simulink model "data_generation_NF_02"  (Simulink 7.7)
settings: Solver=VariableStepDiscrete  StartTime=0.0  StopTime=3000  RelTol=1e-3
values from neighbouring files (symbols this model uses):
  A = [0.9944 -0.1203 -0.4302    [process_model02.m]
  B = [1 0    [process_model02.m]
  C = [1 0 0    [process_model02.m]
  D = zeros(2,2)    [process_model02.m]
  q2 = (0.05)^2    (= 0.0025)    [process_model02.m]    (also in UIO_KF_designs.m)
  r2 = (0.6)^2    (= 0.36)    [process_model02.m]    (also in UIO_KF_designs.m)
  Ts = 0.1    [process_model02.m]
  x0 = [0.01 0.02 0.03]    [process_model02.m]
libraries: simulink x2

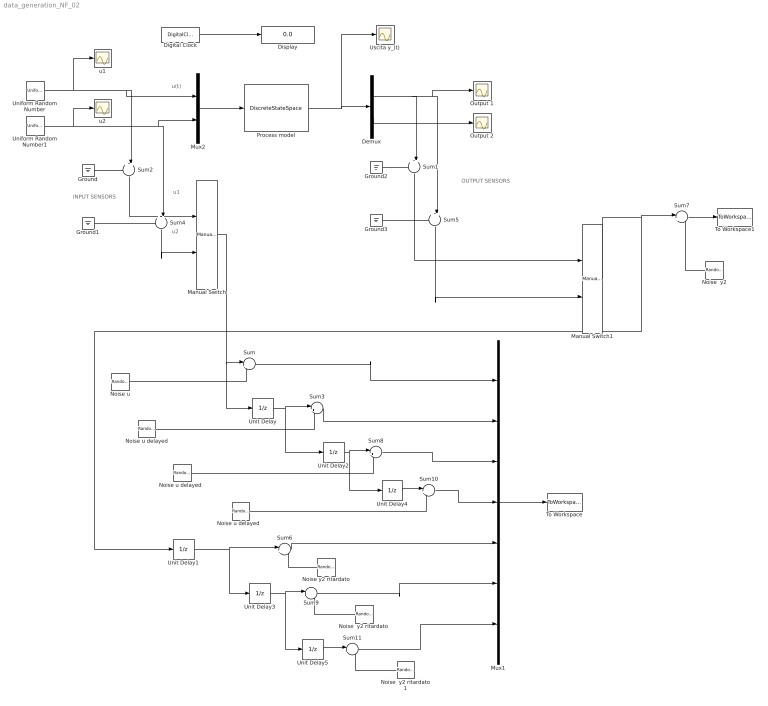
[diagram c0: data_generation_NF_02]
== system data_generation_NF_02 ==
  note: u(t)
  note: INPUT SENSORS
  note: OUTPUT SENSORS
  note: u1
  note: u2
  Demux : Demux  Outputs=2
  Digital Clock : DigitalClock  SampleTime=Ts
  Display : Display
  Ground{,1..3} (4 alike) : Ground
  Manual Switch : simulink/Signal Routing/Manual Switch  SystemSampleTime=-1  sw=1  action=0  varsize=off
  Manual Switch1 : simulink/Signal Routing/Manual Switch  SystemSampleTime=-1  sw=1  action=0  varsize=off
  Mux1 : Mux  Inputs=7
  Mux2 : Mux  Inputs=2
  Noise u : RandomNumber  Variance=q2  Seed=1  SampleTime=Ts
  Noise u delayed : RandomNumber  Variance=q2  Seed=2  SampleTime=Ts
  "Noise u delayed  " : RandomNumber  Variance=q2  Seed=17  SampleTime=Ts
  "Noise u delayed   " : RandomNumber  Variance=q2  Seed=33  SampleTime=Ts
  Noise  y2 : RandomNumber  Variance=r2  Seed=3  SampleTime=Ts
  "Noise  y2 ritardato " : RandomNumber  Variance=r2  Seed=21  SampleTime=Ts
  Noise  y2 ritardato 1 : RandomNumber  Variance=r2  Seed=44  SampleTime=Ts
  Noise y2 ritardato : RandomNumber  Variance=r2  Seed=4  SampleTime=Ts
  Output 1 : Scope
  Output 2 : Scope
  Process model : DiscreteStateSpace  A=A  B=B  C=C  D=D  X0=x0  SampleTime=Ts
  Sum{,3,6..11} (8 alike) : Sum  Inputs=|++
  Sum{1..2,4..5} (4 alike) : Sum  Inputs=++|
  To Workspace : ToWorkspace  VariableName=Psim  SampleTime=Ts  SaveFormat=Array
  To Workspace1 : ToWorkspace  VariableName=Tsim  SampleTime=Ts  SaveFormat=Array
  Uniform Random Number : UniformRandomNumber  Seed=11  SampleTime=Ts
  Uniform Random Number1 : UniformRandomNumber  Minimum=-0.5  Maximum=0.5  Seed=13  SampleTime=Ts
  Unit Delay{,1..5} (6 alike) : UnitDelay  SampleTime=Ts
  Uscita y_(t) : Scope
  u1 : Scope
  u2 : Scope
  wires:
  Digital Clock/1 -> Display/1
  Mux2/1 -> Process model/1
  Uniform Random Number/1 -> u1/1, Mux2/1, Sum2/2
  Process model/1 -> Uscita y_(t)/1, Demux/1
  Uniform Random Number1/1 -> u2/1, Mux2/2, Sum4/2
  Demux/1 -> Output 1/1, Sum5/2, Sum1/2
  Demux/2 -> Output 2/1
  Sum2/1 -> Manual Switch/1
  Sum4/1 -> Manual Switch/2
  Ground/1 -> Sum2/1
  Ground1/1 -> Sum4/1
  Manual Switch/1 -> Sum/1, Unit Delay/1
  Unit Delay/1 -> Sum3/1, Unit Delay2/1
  Noise u/1 -> Sum/2
  Noise u delayed/1 -> Sum3/2
  Sum1/1 -> Manual Switch1/1
  Sum5/1 -> Manual Switch1/2
  Unit Delay1/1 -> Sum6/1, Unit Delay3/1
  Noise y2 ritardato/1 -> Sum6/2
  Manual Switch1/1 -> Unit Delay1/1, Sum7/1
  Ground2/1 -> Sum1/1
  Ground3/1 -> Sum5/1
  Sum7/1 -> To Workspace1/1
  Noise  y2/1 -> Sum7/2
  Unit Delay2/1 -> Sum8/1, Unit Delay4/1
  "Noise u delayed  "/1 -> Sum8/2
  Mux1/1 -> To Workspace/1
  Unit Delay3/1 -> Sum9/1, Unit Delay5/1
  "Noise  y2 ritardato "/1 -> Sum9/2
  Unit Delay4/1 -> Sum10/1
  "Noise u delayed   "/1 -> Sum10/2
  Sum6/1 -> Mux1/5
  Sum10/1 -> Mux1/4
  Sum8/1 -> Mux1/3
  Sum3/1 -> Mux1/2
  Sum/1 -> Mux1/1
  Unit Delay5/1 -> Sum11/1
  Noise  y2 ritardato 1/1 -> Sum11/2
  Sum11/1 -> Mux1/7
  Sum9/1 -> Mux1/6
